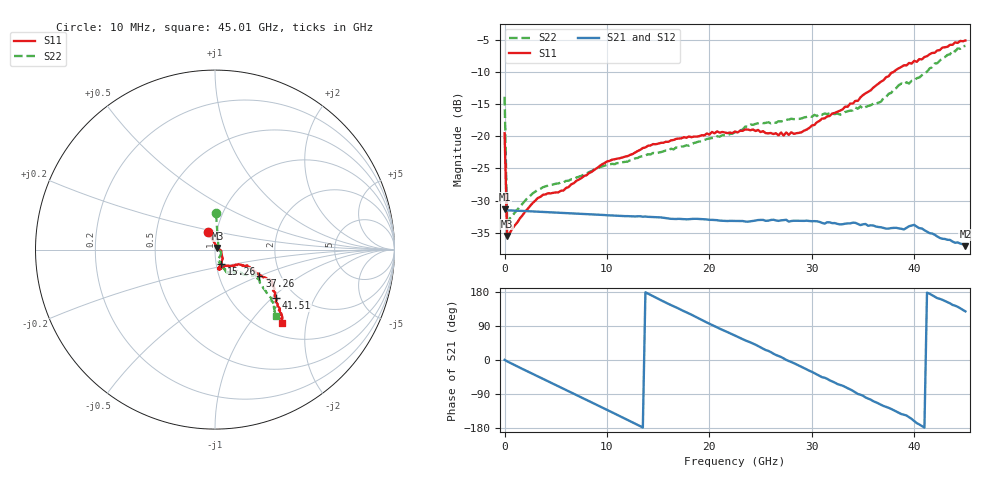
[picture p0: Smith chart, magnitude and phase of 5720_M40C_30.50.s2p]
! Device:  ADRF5720
! Description: 0.5dB LSB GaAs MMIC 6-bit Digital Attenuator
! Frequency:  0.000009 -  40 GHz
! Ports:
!	RF1	= Port 1
!	RF2	= Port 2
! Vdd:  3.3 Volt
! Vss:  -3.3 Volt
! Control:  0/3.3 Volt
! State:  30.50 dB attenuation
! Data:  The device was measured using G-S-G Probes on a matrix board.
!  Data was collected using an calibrated 4 port network analyzer.
!  The reference plane for this measurement is at the launchers.
! Note:  Analog Devices supplies this data as a sample of measured data
!  for this product.  Your particular data for this product may vary.
!  Data was taken at -40 degrees C.
!  Analog Devices reserves the right to change this data at anytime.
# GHZ S DB R 45.0
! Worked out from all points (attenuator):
!   181 points, 10 MHz to 45.01 GHz, reference 45 ohm
!   highest |S21| = -31.32 dB at 10 MHz (marker M1); lowest = -37.1 dB at 45.01 GHz (marker M2)
!   lowest |S11| = -35.5 dB at 260 MHz (marker M3), VSWR 1.03, Z = 46.3 + j0.883 ohm
!   |S11| at or under -10 dB: start of sweep to 38.01 GHz
!   |S22| runs from -33.6 to -6.0 dB; largest |S21 - S12| = 0.00021
!   S11 on the Smith chart (normalised r, x): 10 MHz: 0.91, +0.18; 15.26 GHz: 1.06, -0.17; 37.26 GHz: 1.56, -0.50; 41.51 GHz: 1.60, -1.06; 45.01 GHz: 1.24, -1.47
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0.01  -19.53 112.3  -31.32 0.5  -31.34 0.4  -13.86 88.4
0.26  -35.50 34.6  -31.51 -3.6  -31.53 -3.7  -33.56 23.1
2.01  -31.72 1.1  -31.62 -26.9  -31.65 -27.0  -30.01 -16.1
3.26  -29.59 -8.9  -31.72 -43.4  -31.74 -43.4  -28.28 -28.5
5.76  -28.43 -25.0  -31.91 -76.0  -31.93 -76.0  -27.15 -47.9
7.76  -26.19 -39.2  -32.08 -102.1  -32.10 -102.1  -25.94 -62.1
10.01  -23.91 -48.2  -32.28 -131.6  -32.30 -131.6  -24.47 -68.2
15.26  -21.03 -66.5  -32.61 158.1  -32.63 158.0  -22.47 -70.5
20.26  -19.33 -77.8  -32.99 92.5  -33.01 92.5  -20.27 -64.6
22.76  -19.41 -80.2  -33.17 61.3  -33.19 61.3  -19.31 -65.4
24.01  -19.06 -75.2  -33.22 46.5  -33.23 46.5  -18.20 -64.0
27.26  -19.89 -65.7  -33.03 4.3  -33.04 4.1  -17.65 -62.0
30.26  -18.24 -47.1  -33.19 -34.5  -33.21 -34.6  -16.68 -61.9
32.76  -16.02 -31.4  -33.70 -65.7  -33.71 -65.8  -16.65 -55.5
34.51  -14.50 -29.4  -33.62 -89.6  -33.63 -89.7  -15.73 -48.7
37.26  -10.82 -30.5  -34.35 -123.7  -34.36 -123.8  -13.93 -41.8
37.76  -10.16 -30.0  -34.27 -129.1  -34.31 -129.2  -13.27 -40.0
38.76  -9.22 -28.5  -34.38 -142.7  -34.40 -142.9  -11.80 -35.0
40.01  -8.28 -31.6  -33.77 -160.9  -33.83 -160.9  -11.33 -32.5
41.51  -7.27 -38.3  -35.06 174.9  -35.06 175.1  -9.46 -37.9
43.76  -5.78 -43.9  -36.37 145.3  -36.41 145.4  -6.64 -43.7
45.01  -5.11 -47.6  -37.08 128.3  -37.17 128.2  -5.96 -47.6
